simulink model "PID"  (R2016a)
settings: Solver=VariableStepAuto  StartTime=0.0  StopTime=10.0  RelTol=1e-3
libraries: vexarmcortexlib x4, simulink x1

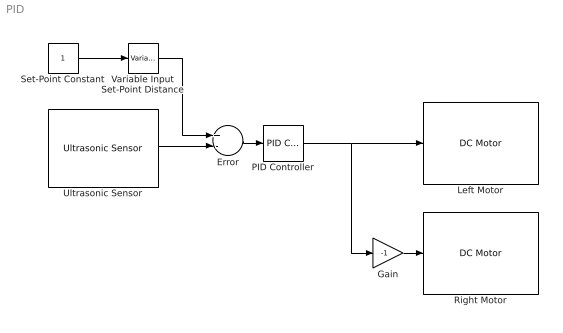
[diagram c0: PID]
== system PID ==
  Error : Sum  Inputs=+-
  Gain : Gain  Gain=-1
  Left Motor : vexarmcortexlib/DC Motor  motor=3  scaleFactor=1/13.5  SimulationOut=off
  PID Controller : simulink/Continuous/PID Controller  Controller=PID  TimeDomain=Continuous-time  SampleTime=-1  IntegratorMethod=Forward Euler  FilterMethod=Forward Euler  Form=Parallel  UseFilter=on  ControllerParametersSource=internal  P=40  I=1  D=0  N=100  InitialConditionSource=internal  InitialConditionForIntegrator=0  InitialConditionForFilter=0  ExternalReset=none  LimitOutput=off  UpperSaturationLimit=inf  LowerSaturationLimit=-inf  LinearizeAsGain=on  AntiWindupMode=none  Kb=1  TrackingMode=off  Kt=1  PParamMin=[]  PParamMax=[]  IParamMin=[]  IParamMax=[]  DParamMin=[]  DParamMax=[]  NParamMin=[]  NParamMax=[]  KbParamMin=[]  KbParamMax=[]  KtParamMin=[]  KtParamMax=[]  POutMin=[]  POutMax=[]  IOutMin=[]  IOutMax=[]  DOutMin=[]  DOutMax=[]  NOutMin=[]  NOutMax=[]  KbOutMin=[]  KbOutMax=[]  KtOutMin=[]  KtOutMax=[]  IntegratorOutMin=[]  IntegratorOutMax=[]  FilterOutMin=[]  FilterOutMax=[]  SumOutMin=[]  SumOutMax=[]  SumI1OutMin=[]  SumI1OutMax=[]  SumI2OutMin=[]  SumI2OutMax=[]  SumI3OutMin=[]  SumI3OutMax=[]  SumDOutMin=[]  SumDOutMax=[]  SaturationOutMin=[]  SaturationOutMax=[]  IntegratorContinuousStateAttributes=''  IntegratorStateMustResolveToSignalObject=off  IntegratorRTWStateStorageClass=Auto  FilterContinuousStateAttributes=''  FilterStateMustResolveToSignalObject=off  FilterRTWStateStorageClass=Auto  DifferentiatorICPrevScaledInput=0  DifferentiatorOutMin=[]  DifferentiatorOutMax=[]
  Right Motor : vexarmcortexlib/DC Motor  motor=3  scaleFactor=1/13.5  SimulationOut=off
  Set-Point Constant : Constant
  Ultrasonic Sensor : vexarmcortexlib/Ultrasonic Sensor  inputPin=3  outputPin=2  inputPortSim=off  SampleTime=0.2
  Variable Input Set-Point Distance : vexarmcortexlib/Utilities/Variable Input  low=0  gain=0.2  high=2
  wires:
  PID Controller/1 -> Gain/1, Left Motor/1
  Error/1 -> PID Controller/1
  Ultrasonic Sensor/1 -> Error/2
  Set-Point Constant/1 -> Variable Input Set-Point Distance/1
  Variable Input Set-Point Distance/1 -> Error/1
  Gain/1 -> Right Motor/1
